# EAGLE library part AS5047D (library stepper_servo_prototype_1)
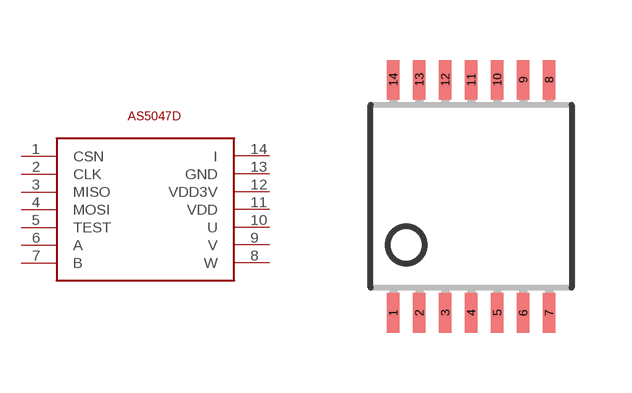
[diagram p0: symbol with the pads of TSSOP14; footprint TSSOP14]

Designator prefix -

## AS5047D  [TSSOP14]
1  CSN
2  CLK
3  MISO
4  MOSI
5  TEST
6  A
7  B
8  W
9  V
10  U
11  VDD
12  VDD3V
13  GND
14  I

## Footprint TSSOP14 (pad centres in mm)
Thin Shrink Small Outline Plastic 14
smd 0.305 x 0.991: 1 -1.95,-2.918; 2 -1.3,-2.918; 3 -0.65,-2.918; 4 0,-2.918; 5 0.65,-2.918; 6 1.3,-2.918; 7 1.95,-2.918; 8 1.95,2.918; 9 1.3,2.918; 10 0.65,2.918; 11 0,2.918; 12 -0.65,2.918; 13 -1.3,2.918; 14 -1.95,2.918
